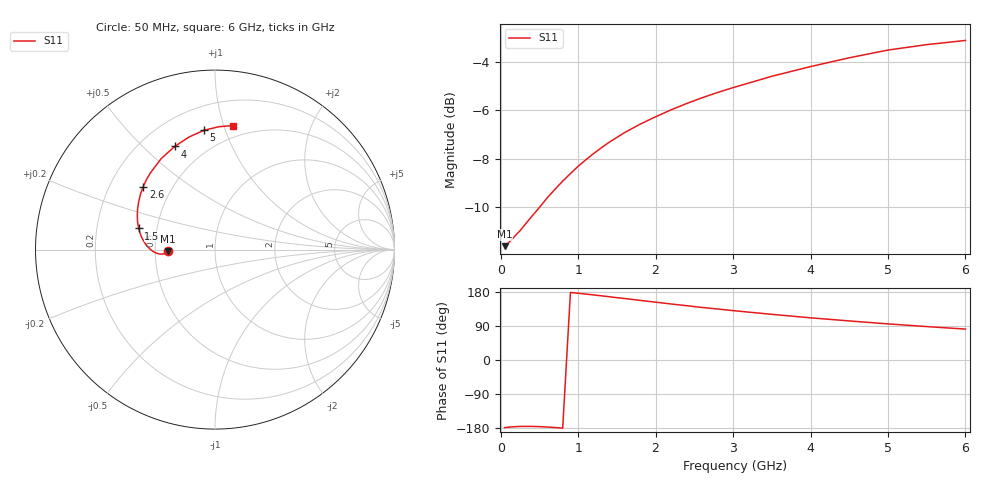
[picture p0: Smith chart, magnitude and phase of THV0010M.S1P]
! SIEMENS Discrete & RF Semiconductors
! BAS70
! Si Schottky Diode in SOT23
! IF = 10 mA
! S-Parameters:  February  1997
# GHz  S  MA  R  50
!  f  S11
! GHz  MAG  ANG
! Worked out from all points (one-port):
!   34 points, 50 MHz to 6 GHz, reference 50 ohm
!   lowest |S11| = -11.6 dB at 50 MHz (marker M1), VSWR 1.71, Z = 29.2 - j0.431 ohm
!   |S11| at or under -10 dB: start of sweep to 503 MHz
!   S11 on the Smith chart (normalised r, x): 50 MHz: 0.58, -0.01; 1.5 GHz: 0.39, +0.12; 2.6 GHz: 0.34, +0.34; 4 GHz: 0.34, +0.63; 5 GHz: 0.35, +0.85; 6 GHz: 0.40, +1.08
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0.05  0.2626 -178.5
0.1  0.2669 -177.3
0.2  0.2774 -175.7
0.25  0.2827 -175.3
0.4  0.3025 -175.2
0.5  0.3158 -175.8
0.6  0.3305 -176.8
0.7  0.3442 -178.2
0.8  0.3579 -179.9
0.9  0.3709 178.2
1  0.3841 176.2
1.2  0.4081 171.7
1.4  0.4305 167.0
1.5  0.4405 164.5
1.6  0.4508 162.2
1.8  0.4691 157.3
2  0.486 152.6
2.2  0.5023 147.8
2.4  0.5176 143.3
2.6  0.532 138.7
2.8  0.5456 134.5
3  0.5582 130.3
3.5  0.5892 120.5
4  0.6171 111.3
4.5  0.6434 103.1
5  0.6675 95.3
5.5  0.685 88.2
6  0.6987 81.6
